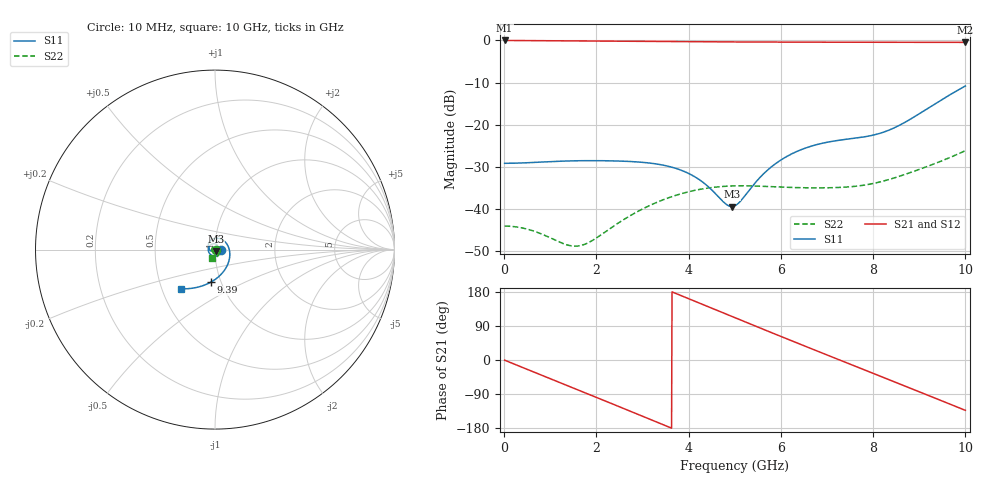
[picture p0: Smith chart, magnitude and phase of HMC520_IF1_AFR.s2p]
! Analog Devices, Inc.
! 1 Analog Way
! Wilmington, MA 01887
! http://www.analog.com
! Date:  2021-09-07 NN
! Board Name:  EV1HMC520ALC4 Revision A with HMC520ALC4 installed
! File Description:  Automatic Fixture Removal S-Parameters for IF1 Port connector and board loss de-embedding
! File Generation:  Calibrated Network Analyzer
! Chip Part Number:  HMC520A
! Chip Description:  GaAs, MMIC, IQ Mixer
! Chip Frequency:  6 to 10 GHz
! Chip Package:  LCC, 3.9 x 3.9 x 0.9 mm
! IF1 Port:  HMC520ALC4 removed and end of trace left open
!Note:
!  Analog Devices supplies this data as a sample of measured data at the evaluation board
!  ports for this product.  Your particular data for this product may vary.
!  Analog Devices reserves the right to change this data at anytime.
!  All lines below in this file are as is from the Network Analyzer.
!Agilent Technologies,N5245A,MY52451809,A.10.47.06
!Automatic Fixture Removal (AFR)
!Date: Friday, August 27, 2021 5:03:12 AM
!S2P File: Measurements: S11,S21,S12,S22:
# MHz S  RI  R 50
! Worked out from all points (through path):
!   1000 points, 10 MHz to 10 GHz, reference 50 ohm
!   highest |S21| = 0.00 dB at 10 MHz (marker M1); lowest = -0.5 dB at 10 GHz (marker M2)
!   group delay of S21, straight-line fit = 137 ps
!   lowest |S11| = -39.4 dB at 4.94 GHz (marker M3), VSWR 1.02, Z = 50.4 - j0.977 ohm
!   |S11| at or under -10 dB: start of sweep to end of sweep
!   |S22| runs from -48.9 to -26.2 dB; largest |S21 - S12| = 1.4e-15
!   S11 on the Smith chart (normalised r, x): 10 MHz: 1.07, -0.00; 9.39 GHz: 0.89, -0.34; 10 GHz: 0.63, -0.30
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10  0.0348 -0.000505  0.9999 -0.00859  0.9999 -0.00859  0.00625 -8.15e-05
750  0.0171 -0.0315  0.7928 -0.5959  0.7928 -0.5959  0.00267 -0.00445
1230  -0.00592 -0.0363  0.4846 -0.8597  0.4846 -0.8597  -0.00122 -0.00378
1680  -0.0258 -0.027  0.1231 -0.976  0.1231 -0.976  -0.00362 -0.000725
2060  -0.0357 -0.0111  -0.1975 -0.9608  -0.1975 -0.9608  -0.00386 0.00276
2440  -0.0363 0.00732  -0.4958 -0.8429  -0.4958 -0.8429  -0.00224 0.0062
2910  -0.0249 0.026  -0.7865 -0.5747  -0.7865 -0.5747  0.00225 0.00913
3340  -0.0075 0.033  -0.9387 -0.2463  -0.9387 -0.2463  0.00812 0.00904
3710  0.00711 0.0296  -0.9655 0.064  -0.9655 0.064  0.0132 0.00582
4090  0.0165 0.0185  -0.8895 0.374  -0.8895 0.374  0.0164 -0.000583
4940  0.00445 -0.00969  -0.4014 0.872  -0.4014 0.872  0.0077 -0.0171
5010  0.00164 -0.0108  -0.3474 0.8945  -0.3474 0.8945  0.00599 -0.0178
5400  -0.0159 -0.0107  -0.0307 0.9574  -0.0307 0.9574  -0.00454 -0.0182
5800  -0.0317 0.00138  0.295 0.9099  0.295 0.9099  -0.0139 -0.012
6670  -0.0261 0.0493  0.8317 0.4676  0.8317 0.4676  -0.0144 0.0104
7080  0.000258 0.063  0.9406 0.1553  0.9406 0.1553  -0.00675 0.0165
7480  0.0341 0.0585  0.9381 -0.1662  0.9381 -0.1662  0.00167 0.0182
7890  0.066 0.031  0.8252 -0.475  0.8252 -0.475  0.00988 0.0168
8340  0.0826 -0.0239  0.589 -0.7472  0.589 -0.7472  0.0189 0.0118
8870  0.0579 -0.1072  0.2053 -0.9281  0.2053 -0.9281  0.0276 -0.00268
9390  -0.024 -0.1819  -0.2126 -0.9258  -0.2126 -0.9258  0.023 -0.0269
10000  -0.1876 -0.2185  -0.6463 -0.6951  -0.6463 -0.6951  -0.0152 -0.0468
